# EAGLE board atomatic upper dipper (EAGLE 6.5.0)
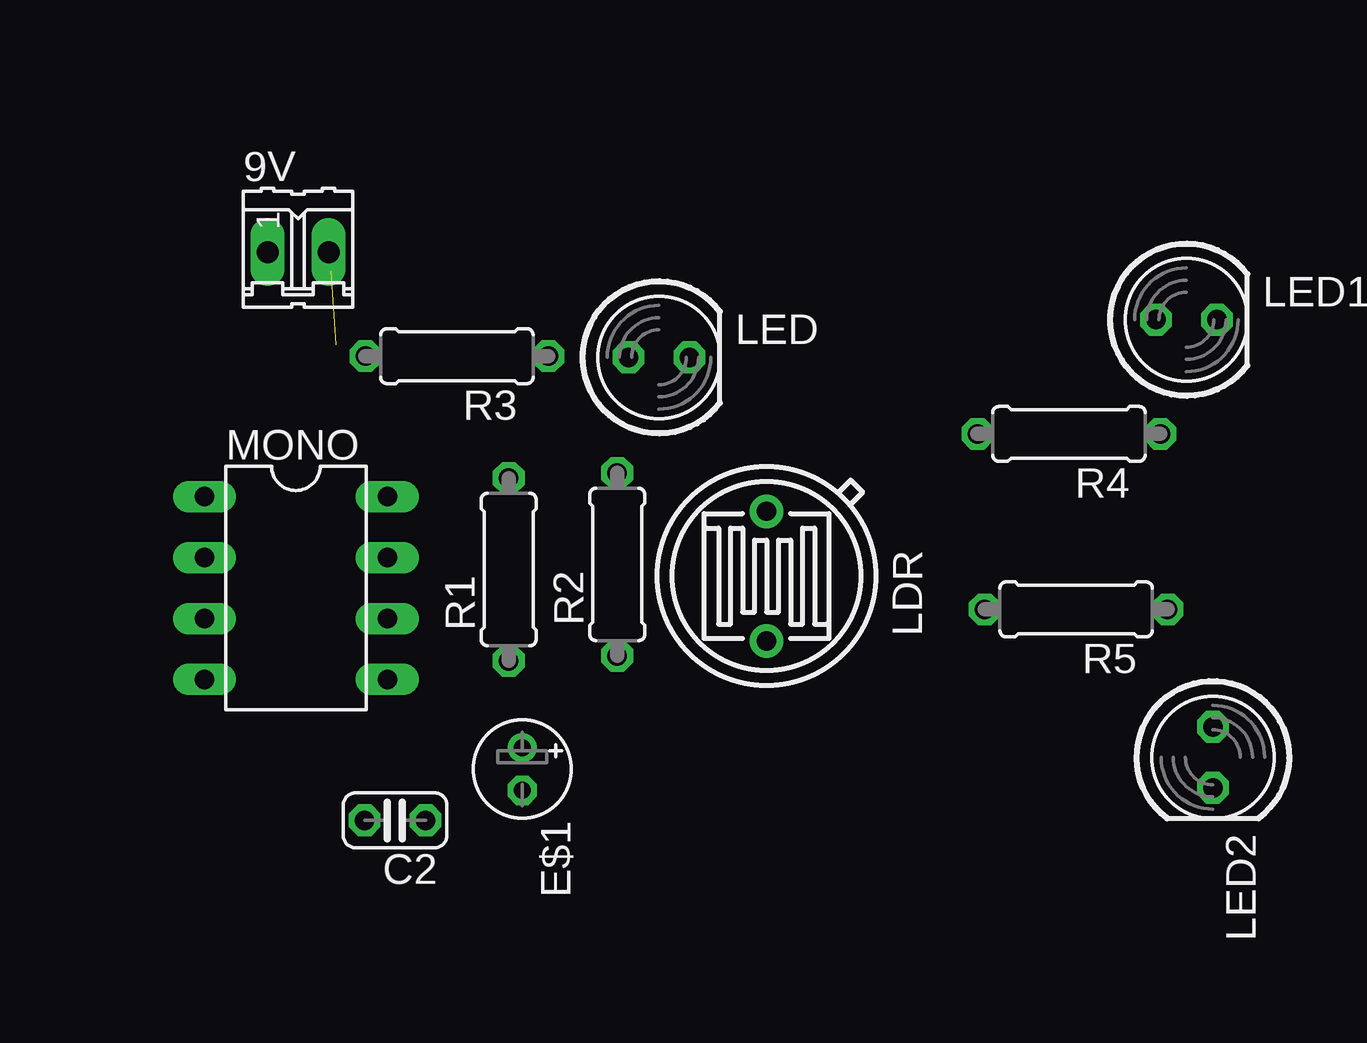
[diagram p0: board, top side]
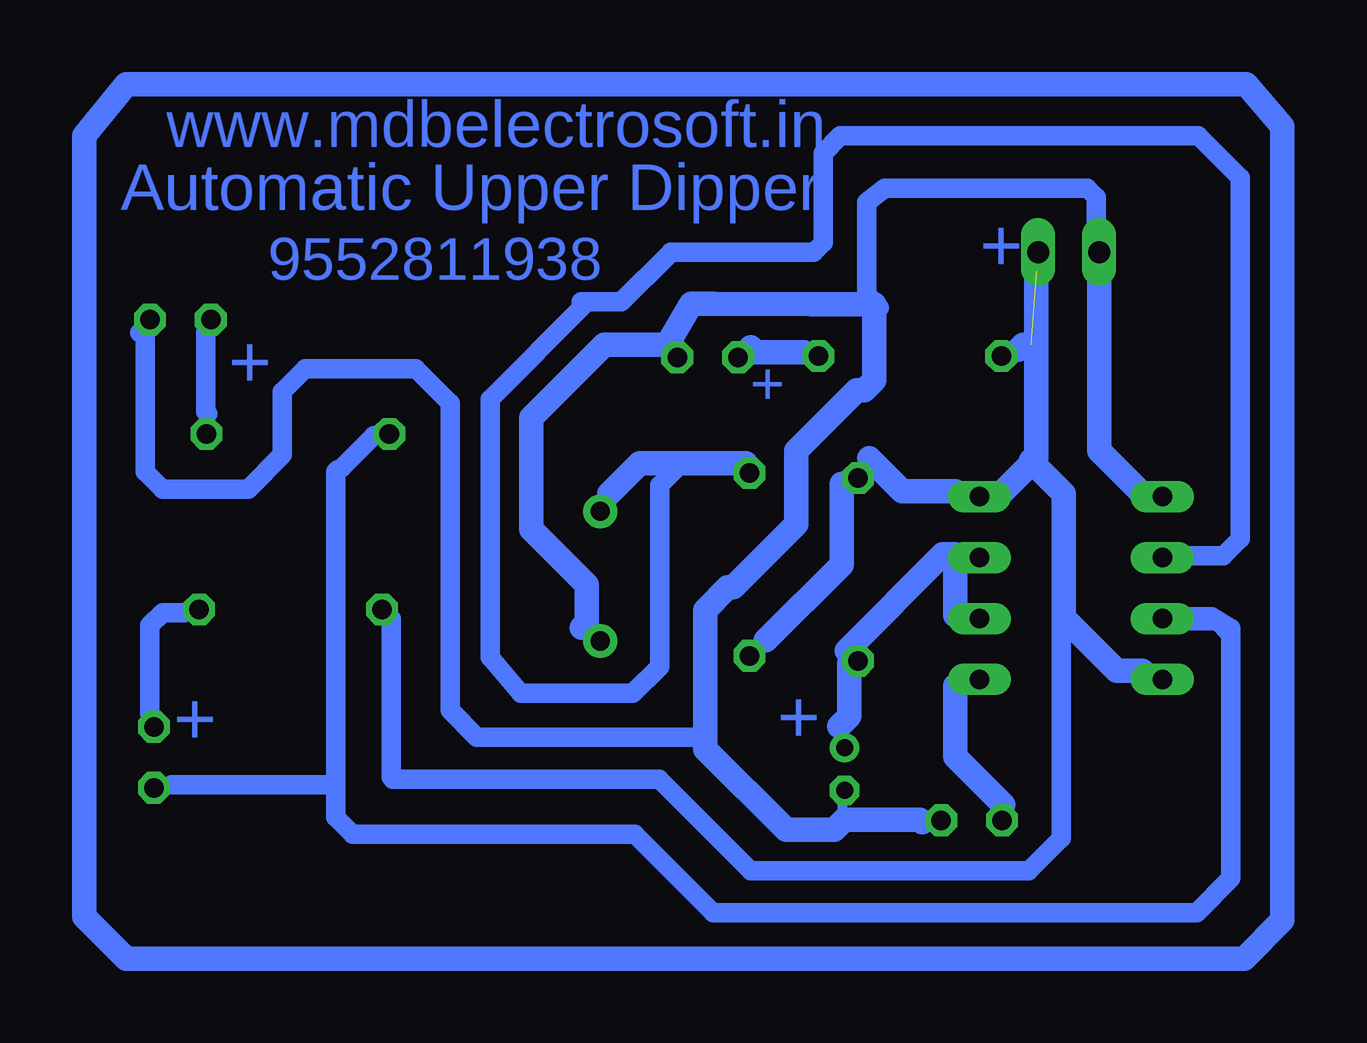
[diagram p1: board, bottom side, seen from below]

No outline drawn. Coordinates in mm, seen from the top.
Copper layers (1*16): Top 0.035mm / dielectric 1.5mm / Bottom 0.035mm
Design rules "default": minimum track width 10mil, minimum drill 24mil, track to track 8mil, track to pad 8mil, pad to pad 8mil, via to via 8mil, smd to smd 8mil, copper to edge 40mil, drill to drill 8mil, minimum pad ring 10mil, minimum via ring 8mil, stop-mask expansion 4mil, vias tented up to drill 0mil, thermal gap 10mil

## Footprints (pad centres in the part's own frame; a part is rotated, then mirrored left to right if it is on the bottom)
02P = drill 0.914 long: 1 -1.27,0; 2 1.27,0
C025-024X044 = drill 0.813 octagon: 1 -1.27,0; 2 1.27,0
E1,8-4 = drill 0.711 pad 1.168: + -0.889,0 | drill 0.711 pad 1.168 octagon: - 0.889,0
TO-5_V10 = drill 0.8 pad 1.4: 1 -2.7,0; 2 2.7,0
LED5MM = drill 0.813 octagon: A -1.27,0; K 1.27,0
DIL08 = drill 0.813 long: 1 -3.81,-3.81; 2 -1.27,-3.81; 3 1.27,-3.81; 4 3.81,-3.81; 5 3.81,3.81; 6 1.27,3.81; 7 -1.27,3.81; 8 -3.81,3.81
0207/7 = drill 0.813 octagon: 1 -3.81,0; 2 3.81,0

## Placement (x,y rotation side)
9V  [02P]  21.68,50.82 0 top
C2  0.1uf  [C025-024X044]  25.72,27.15 180 top
E$1  [E1,8-4]  31.02,29.29 270 top
LDR  [TO-5_V10]  41.2,37.33 90 top
LED  [LED5MM]  36.72,46.44 0 top
LED1  [LED5MM]  58.69,48.01 0 top
LED2  [LED5MM]  59.8,29.78 270 top
MONO  IC555  [DIL08]  21.59,36.83 270 top
R1  330  [0207/7]  30.45,37.6 90 top
R2  47k  [0207/7]  34.98,37.82 90 top
R3  330  [0207/7]  28.3,46.49 180 top
R4  330  [0207/7]  53.8,43.25 180 top
R5  330  [0207/7]  54.1,35.94 180 top

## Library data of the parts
9V = con-amp-quick
C2 E$1 R1-R5 = rcl
LDR = photo-elements
LED LED1 LED2 = led
MONO = 40xx

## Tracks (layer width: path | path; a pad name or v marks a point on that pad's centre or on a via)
S$1
  Bottom 1.016: 29.98,42.23 28.61,40.86 26.41,40.86
S$2
  Bottom 1.016: 30.83,33.7 30.83,31.49 31.25,31.07
S$3
  Bottom 1.016: 26.41,35.7 26.41,38.23 26.93,38.23 30.93,34.23
S$4
  Bottom 0.813: 37.93,41.91 38.73,41.12 38.73,33.56 39.84,32.45 44.52,32.45 45.79,33.95 45.79,44.69 41.81,48.67
S$5
  Bottom 1.016: 20.41,50.03 20.41,42.55 18.73,40.86
S$6
  Bottom 1.016: 18.62,33.38 19.67,33.38 21.88,35.6 21.88,40.76 23.25,42.13
S$7
  Bottom 0.813: 20.52,51.94 20.52,53.11 20.9,53.5 29.34,53.5 30.1,52.9 30.1,49.04 29.57,48.51
S$8
  Bottom 1.016: 26.41,32.75 26.41,29.8 24.41,27.8
S$9
  Bottom 0.813: 16.98,38.09 16.9,38.17 15.24,38.17 14.52,38.89 14.52,53.92 16.27,55.67 31.19,55.67 31.9,54.95 31.9,51.22 32.3,50.82 38.25,50.82
S$10
  Bottom 0.813: 21.82,35.79 21.98,35.63 21.98,26.4 23.33,25.05 34.92,25.05 38.73,28.87 49.84,28.87 49.92,28.95 49.92,35.55
S$11
  Bottom 1.016: 38.4,46.97 37.41,48.67 36.47,48.67 32.4,48.66 29.77,48.66 29.77,45.5 30.2,45.08 30.51,45.08 33.03,42.55 33.03,39.49 35.67,36.86
S$12
  Bottom 1.016: 32.72,46.66 34.72,46.66 34.93,46.87
S$13
  Bottom 1.016: 31.14,41.18 31.14,37.8 34.3,34.65
S$14
  Bottom 1.016: 35.14,42.02 39.56,42.02 40.82,40.76
S$15
  Bottom 1.016: 38.72,46.97 41.03,46.97 44.08,43.92 44.08,39.28 41.77,36.97 41.77,35.39 41.98,35.18
S$16
  Bottom 0.813: 38.33,50.74 40.32,48.75 41.98,48.75
S$17
  Bottom 0.813: 52.14,41.75 52.22,41.67 52.22,27.28 51.5,26.56 39.76,26.56 36.5,23.3 16.35,23.3 14.92,24.73
S$18
  Bottom 0.813: 50.63,43.18 51.98,41.83
S$19
  Bottom 1.016: 35.77,36.86 35.88,36.86 36.82,35.91 36.82,30.12 33.46,26.75 31.46,26.75 31.04,27.17 27.88,27.17 27.77,27.07
S$20
  Bottom 0.406: 30.95,27.15 31.09,27.15 31.09,27.98
S$21
  Bottom 0.813: 52.3,28.63 59.04,28.63
S$22
  Bottom 0.813: 16.9,35.47 15.48,35.47 14.92,34.91
S$23
  Bottom 0.813: 58.53,35.8 59.43,35.8 59.96,35.28 59.96,31.58
S$24
  Bottom 1.016: 14.29,57.82 60.95,57.82 62.69,55.67 62.69,23.14 60.94,21.39 14.36,21.39 12.78,22.98 12.78,56.07 14.29,57.82
S$25
  Bottom 0.813: 57.63,47.49 57.63,44.17 57.55,44.1
S$26
  Bottom 0.813: 16.9,35.55 16.82,35.63 15.71,35.63 14.92,35.15 14.92,24.73
S$27
  Bottom 0.813: 60.39,47.48 60.15,47.24 60.15,41.67 59.44,40.96 55.87,40.96 54.44,42.38 54.44,45.01 53.48,45.97 48.88,45.97 47.45,44.54 47.45,31.73 46.34,30.62 37.06,30.62
VCC  (1 unrouted)
  Bottom 1.016: 23.25,46.97 23.57,46.97 23.78,46.76 | 23.04,50.03 23.04,42.23 24.51,40.76

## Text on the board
Bottom: www.mdbelectrosoft.in | Automatic Upper Dipper | + | 9552811938 | + | + | + | +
